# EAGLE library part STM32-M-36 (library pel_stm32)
STM32F103 Medium Density 36 Pins
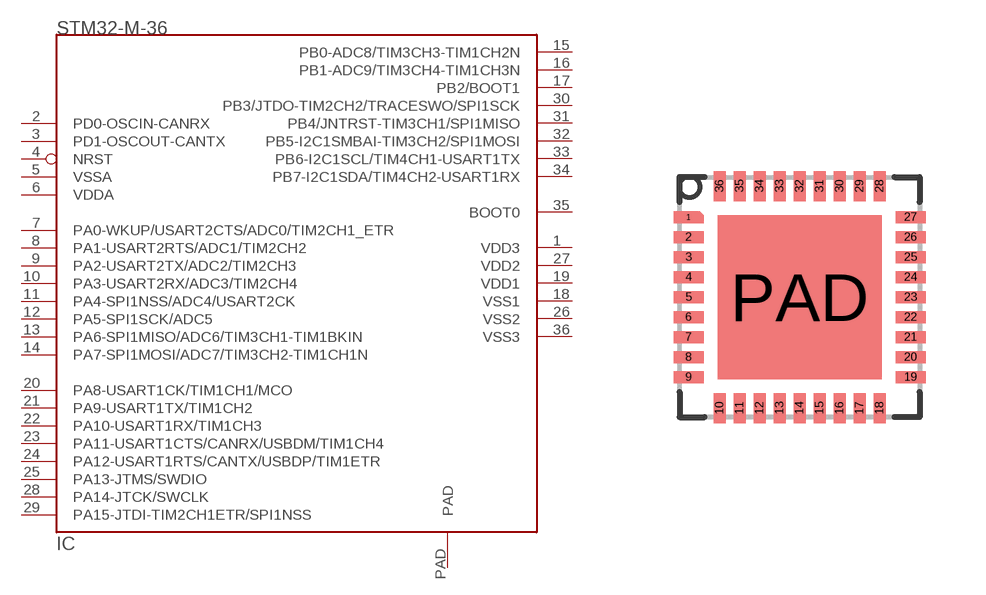
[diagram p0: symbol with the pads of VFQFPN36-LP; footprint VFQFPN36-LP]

Designator prefix IC

## STM32-M-36  [VFQFPN36-LP]
1  VDD3  pwr
2  PD0-OSCIN-CANRX
3  PD1-OSCOUT-CANTX
4  NRST
5  VSSA  pwr
6  VDDA  pwr
7  PA0-WKUP/USART2CTS/ADC0/TIM2CH1_ETR
8  PA1-USART2RTS/ADC1/TIM2CH2
9  PA2-USART2TX/ADC2/TIM2CH3
10  PA3-USART2RX/ADC3/TIM2CH4
11  PA4-SPI1NSS/ADC4/USART2CK
12  PA5-SPI1SCK/ADC5
13  PA6-SPI1MISO/ADC6/TIM3CH1-TIM1BKIN
14  PA7-SPI1MOSI/ADC7/TIM3CH2-TIM1CH1N
15  PB0-ADC8/TIM3CH3-TIM1CH2N
16  PB1-ADC9/TIM3CH4-TIM1CH3N
17  PB2/BOOT1
18  VSS1  pwr
19  VDD1  pwr
20  PA8-USART1CK/TIM1CH1/MCO
21  PA9-USART1TX/TIM1CH2
22  PA10-USART1RX/TIM1CH3
23  PA11-USART1CTS/CANRX/USBDM/TIM1CH4
24  PA12-USART1RTS/CANTX/USBDP/TIM1ETR
25  PA13-JTMS/SWDIO
26  VSS2  pwr
27  VDD2  pwr
28  PA14-JTCK/SWCLK
29  PA15-JTDI-TIM2CH1ETR/SPI1NSS
30  PB3/JTDO-TIM2CH2/TRACESWO/SPI1SCK
31  PB4/JNTRST-TIM3CH1/SPI1MISO
32  PB5-I2C1SMBAI-TIM3CH2/SPI1MOSI
33  PB6-I2C1SCL/TIM4CH1-USART1TX
34  PB7-I2C1SDA/TIM4CH2-USART1RX
35  BOOT0  in
36  VSS3  pwr
PAD  PAD  nc

## Footprint VFQFPN36-LP (pad centres in mm)
smd 0.65 x 0.2: 1 -2.775,2
smd 0.75 x 0.3: 2 -2.775,1.5; 3 -2.775,1; 4 -2.775,0.5; 5 -2.775,0; 6 -2.775,-0.5; 7 -2.775,-1; 8 -2.775,-1.5; 9 -2.775,-2; 19 2.775,-2; 20 2.775,-1.5; 21 2.775,-1; 22 2.775,-0.5; 23 2.775,0; 24 2.775,0.5; 25 2.775,1; 26 2.775,1.5; 27 2.775,2
smd 0.3 x 0.75: 10 -2,-2.775; 11 -1.5,-2.775; 12 -1,-2.775; 13 -0.5,-2.775; 14 0,-2.775; 15 0.5,-2.775; 16 1,-2.775; 17 1.5,-2.775; 18 2,-2.775; 28 2,2.775; 29 1.5,2.775; 30 1,2.775; 31 0.5,2.775; 32 0,2.775; 33 -0.5,2.775; 34 -1,2.775; 35 -1.5,2.775; 36 -2,2.775
smd 4.1 x 4.1: PAD 0,0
